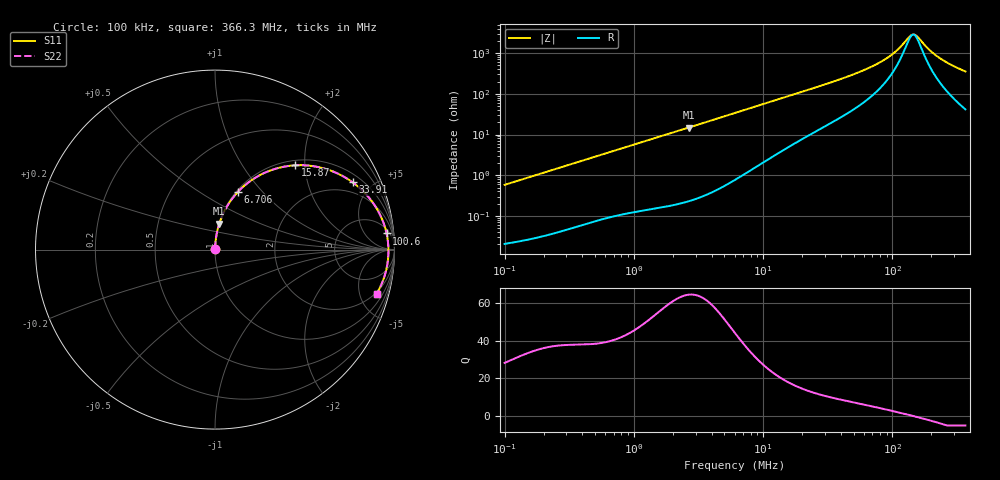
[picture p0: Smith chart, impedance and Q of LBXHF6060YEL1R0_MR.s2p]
! LBXHF6060YEL1R0_MR  S-PARAMETER MODEL  ( General Type )
! Model Generated by TAIYO YUDEN Corporation (http://www.ty-top.com)
! Version 1.0
! TAIYO YUDEN Control No. 200120NI43SB-FBB
! Copyright(c) 2020 TAIYO YUDEN CO.,LTD. All Rights Reserved.
! Product Description (link to TY-COMPAS)
! https://ds.yuden.co.jp/TYCOMPAS/or/detail?pn=LBXHF6060YEL1R0NMR&u=M
! Products Name : Inductors
! Characteristics :
!  Inductance : 1.0 uH , SRF(min) : 90 MHz , DC Resistance(max) : 0.013 Ohm
!  Rated Current : Saturation :13500 mA , Temp Rise : 4000 mA
!  Case Size : 6.0 x 6.0 / 0.236 x 0.236 [mm/inch] , Thickness : 4.5 / 0.177 [mm/inch]
!  (Conditions: Temperature = 25 degC , DC Bias Current/Voltage = 0A / 0V)
! External Node Assignments :
!  1  o---GGG---o  2
! GND o---------o GND
! Frequency Range : 0.1MHz  -  366.261039MHz  [ 402 STEP ]
# MHz S RI R 50
! Freq[MHz].  S11 Real  S11 Imag  S21 Real  S21 Imag  S12 Real  S12 Imag  S22 Real  S22 Imag
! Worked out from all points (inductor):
!   401 points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, 100 kHz to 366.3 MHz, reference 50 ohm
!   read as one part in series: L = 921 nH near 104.2 kHz
!   highest Q = 64.5 at 2.664 MHz (marker M1), where L = 888 nH
!   self-resonance near 144.9 MHz
!   S11 on the Smith chart (normalised r, x): 100 kHz: 1.00, +0.01; 6.706 MHz: 1.02, +0.75; 15.87 MHz: 1.10, +1.78; 33.91 MHz: 1.39, +3.85; 100.6 MHz: 8, +18; 366.3 MHz: 1.83, -7.03
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0.1  0.000239 0.0058  0.9998 -0.0058  0.9998 -0.0058  0.000239 0.0058
0.395307  0.0011 0.0225  0.9989 -0.0225  0.9989 -0.0225  0.0011 0.0225
1.562679  0.00911 0.0864  0.9909 -0.0864  0.9909 -0.0864  0.00911 0.0864
2.66389  0.0238 0.1448  0.9762 -0.1448  0.9762 -0.1448  0.0238 0.1448
6.177387  0.1122 0.3043  0.8878 -0.3043  0.8878 -0.3043  0.1122 0.3043
6.705679  0.1295 0.3235  0.8705 -0.3235  0.8705 -0.3235  0.1295 0.3235
10.10723  0.2507 0.4152  0.7493 -0.4152  0.7493 -0.4152  0.2507 0.4152
15.87233  0.4449 0.4695  0.5551 -0.4695  0.5551 -0.4695  0.4449 0.4695
23.92381  0.6343 0.4437  0.3657 -0.4437  0.3657 -0.4437  0.6343 0.4437
33.90716  0.7674 0.3745  0.2326 -0.3745  0.2326 -0.3745  0.7674 0.3745
61.47043  0.9072 0.218  0.0928 -0.218  0.0928 -0.218  0.9072 0.218
78.6285  0.9375 0.1528  0.0625 -0.1528  0.0625 -0.1528  0.9375 0.1528
94.57258  0.9523 0.1055  0.0477 -0.1055  0.0477 -0.1055  0.9523 0.1055
100.5758  0.9559 0.09  0.0441 -0.09  0.0441 -0.09  0.9559 0.09
113.7498  0.9615 0.0594  0.0385 -0.0594  0.0385 -0.0594  0.9615 0.0594
136.8157  0.9659 0.014  0.0341 -0.014  0.0341 -0.014  0.9659 0.014
148.5162  0.9664 -0.00606  0.0336 0.00606  0.0336 0.00606  0.9664 -0.00606
157.9437  0.9661 -0.0212  0.0339 0.0212  0.0339 0.0212  0.9661 -0.0212
193.9085  0.9617 -0.0723  0.0383 0.0723  0.0383 0.0723  0.9617 -0.0723
223.8532  0.955 -0.1091  0.045 0.1091  0.045 0.1091  0.955 -0.1091
280.5224  0.9371 -0.1694  0.0629 0.1694  0.0629 0.1694  0.9371 -0.1694
366.261  0.9014 -0.2449  0.0986 0.2449  0.0986 0.2449  0.9014 -0.2449
